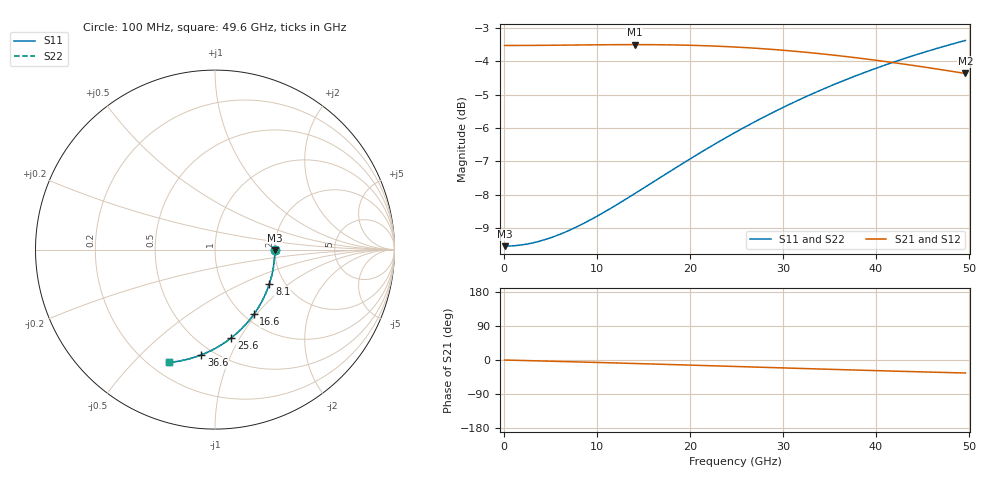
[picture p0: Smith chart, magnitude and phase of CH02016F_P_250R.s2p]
# GHz S RI R 250
! S-Parameters data
! Freq  reS11  imS11  reS21  imS21  reS12  imS12  reS22  imS22
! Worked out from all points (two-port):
!   100 points, 100 MHz to 49.6 GHz, reference 250 ohm
!   highest |S21| = -3.50 dB at 14.1 GHz (marker M1); lowest = -4.4 dB at 49.6 GHz (marker M2)
!   |S21| within 3 dB of the highest: start of sweep to end of sweep
!   lowest |S11| = -9.5 dB at 100 MHz (marker M3), VSWR 2.00, Z = 500 - j2.71 ohm
!   |S11| at or under -10 dB: nowhere
!   |S22| runs from -9.5 to -3.4 dB; largest |S21 - S12| = 0
!   S11 on the Smith chart (normalised r, x): 100 MHz: 2.00, -0.01; 8.1 GHz: 1.67, -0.73; 16.6 GHz: 1.11, -0.97; 25.6 GHz: 0.70, -0.92; 36.6 GHz: 0.43, -0.78; 49.6 GHz: 0.27, -0.64
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0.1  0.3333 -0.00241  0.6667 -0.000732  0.6667 -0.000732  0.3333 -0.00241
2.1  0.3312 -0.0505  0.6666 -0.0154  0.6666 -0.0154  0.3312 -0.0505
4.1  0.3254 -0.0981  0.6663 -0.0301  0.6663 -0.0301  0.3254 -0.0981
6.1  0.3159 -0.1448  0.6659 -0.0451  0.6659 -0.0451  0.3159 -0.1448
8.1  0.3031 -0.1902  0.6651 -0.0603  0.6651 -0.0603  0.3031 -0.1902
8.6  0.2993 -0.2012  0.6648 -0.0641  0.6648 -0.0641  0.2993 -0.2012
11.1  0.2779 -0.2549  0.6631 -0.0836  0.6631 -0.0836  0.2779 -0.2549
14.1  0.2466 -0.3148  0.6599 -0.1075  0.6599 -0.1075  0.2466 -0.3148
16.6  0.2166 -0.3605  0.656 -0.1278  0.656 -0.1278  0.2166 -0.3605
18.6  0.1907 -0.3943  0.652 -0.1441  0.652 -0.1441  0.1907 -0.3943
20.6  0.1633 -0.4254  0.6472 -0.1604  0.6472 -0.1604  0.1633 -0.4254
22.6  0.1347 -0.4539  0.6414 -0.1766  0.6414 -0.1766  0.1347 -0.4539
25.1  0.0979 -0.486  0.633 -0.1965  0.633 -0.1965  0.0979 -0.486
25.6  0.0904 -0.4919  0.6312 -0.2004  0.6312 -0.2004  0.0904 -0.4919
29.1  0.0375 -0.5292  0.6168 -0.227  0.6168 -0.227  0.0375 -0.5292
31.1  0.00712 -0.5473  0.6075 -0.2415  0.6075 -0.2415  0.00712 -0.5473
33.1  -0.0232 -0.5632  0.5976 -0.2554  0.5976 -0.2554  -0.0232 -0.5632
36.6  -0.0756 -0.5863  0.5788 -0.2779  0.5788 -0.2779  -0.0756 -0.5863
39.1  -0.1122 -0.5993  0.5644 -0.2926  0.5644 -0.2926  -0.1122 -0.5993
41.6  -0.148 -0.6097  0.5495 -0.3061  0.5495 -0.3061  -0.148 -0.6097
45.6  -0.2031 -0.6216  0.5249 -0.3252  0.5249 -0.3252  -0.2031 -0.6216
49.6  -0.2553 -0.6285  0.4998 -0.3412  0.4998 -0.3412  -0.2553 -0.6285
